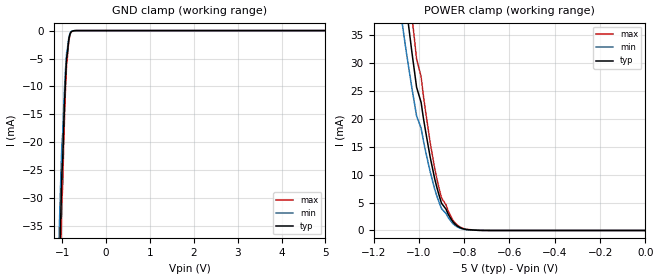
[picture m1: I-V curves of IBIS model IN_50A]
| TEXAS INSTRUMENTS INCORPORATED
| Standard Linear and Logic Group / High Volume Linear
| IBIS Model of TPD6E05U06
| Six Channel ESD Protection Device
| This file contains package information for the following:
|  UQFN 14-pin  package as [Component] TPD6E05U06RVZR
| This device can be powered at the following Vccs:
|  5 volt Vcc
[IBIS Ver]   3.2
[Comment char]  |_char
[File Name]   tpd6e05u06.ibs
[File Rev]   1.1
[Date]   12/10/2015
[Source]   Data created from TI-SPICE simulations at TI-SLL/HVL.
   The following is an IBIS list for the TPD4E05U06.
   Please contact sllibis@ti.com with questions and
   comments concerning SLL IBIS models.
[Notes]   Revision_History:
|  Rev 1.1   12/10/2015
|  - c comp values revised per PL's request
|  Rev 1.0 05/02/2013
[Disclaimer]
| This model is designed as an aid for customers of Texas Instruments.
| TI and its licensors and suppliers make no warranties, either expressed
| or implied, with respect to this  model, including the warranties of
| merchantability or fitness for a particular purpose. The model is
| provided solely on an "as is" basis. The entire risk as to its quality
| and performance is with the customer.
[Copyright]
| (C) Copyright 2013 Texas Instruments Incorporated. All rights reserved.
| Component TPD6E05U06RVZR
[Component]   TPD6E05U06RVZR
[Manufacturer]   Texas Instruments, Inc.
[Package]
|   typ   min   max
R_pkg   0.02313   0.00041   0.06326
L_pkg   0.30296nH   0.01585nH   1.03943nH
C_pkg   0.16466pF   0.07425pF   0.45674pF
[Pin]   signal_name   model_name   R_pin   L_pin   C_pin
1   NC   NC   0.00041   0.01757nH   0.07425pF
2   NC   NC   0.00041   0.01662nH   0.09156pF
3   NC   NC   0.00041   0.01593nH   0.1079pF
4   NC   NC   0.00041   0.01585nH   0.10796pF
5   GND   GND   0.00041   0.01593nH   0.45674pF
6   NC   NC   0.00041   0.01662nH   0.09156pF
7   NC   NC   0.00041   0.01755nH   0.07457pF
8   D3-   IN_50A   0.04552   1.03943nH   0.11983pF
9   D3+   IN_50A   0.06326   0.78248nH   0.16047pF
10   GND   GND   0.00041   0.01593nH   0.45674pF
11   D2-   IN_50A   0.04317   0.49796nH   0.1521pF
12   D2+   IN_50A   0.04311   0.49721nH   0.15259pF
13   D1-   IN_50A   0.04898   0.58006nH   0.14353pF
14   D1+   IN_50A   0.04173   0.71227nH   0.11545pF
| Models and submodels in the file (1): IN_50A (Input)
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[Model]   IN_50A
Model_type  Input
Vinl=0
Vinh=5
| variable   typ   min   max
C_comp   0.31pF   0.21pF   0.61pF
[Temperature Range]   40   100   -40
| Ambient temperature   25   85   -40
[Voltage range]   5   5   5
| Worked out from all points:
|   GND clamp passes 1 mA (typ) near -0.84 V on its own axis
|   POWER clamp passes 1 mA (typ) near -0.84 V on its own axis
[GND Clamp]
| IN_50A
| Voltage   I(typ)   I(min)   I(max)
-5V       -1.23A     -985mA     -1.48A
-1.07V    -45.16mA   -36.1mA    -54.2mA
-1.05V    -38.18mA   -30.5mA    -45.8mA
-1.03V    -31.67mA   -25.3mA    -38mA
-1.02V    -28.68mA   -22.9mA    -34.4mA
-1.01V    -25.62mA   -20.5mA    -30.7mA
-990mV    -22.9mA    -18.3mA    -27.5mA
-950mV    -13.12mA   -10.5mA    -15.7mA
-900mV    -4.871mA   -3.9mA     -5.84mA
-850mV    -1.552mA   -1.24mA    -1.86mA
-790mV    -170.1uA   -136uA     -204uA
5V        247pA      198pA      296pA
[POWER Clamp]
| IN_50A
|Voltage   I(typ)   I(min)   I(max)
-5V       1.23A      985mA      1.48A
-1.07V    45.16mA    36.1mA     54.2mA
-1.05V    38.18mA    30.5mA     45.8mA
-1.03V    31.67mA    25.3mA     38mA
-1.02V    28.68mA    22.9mA     34.4mA
-1.01V    25.62mA    20.5mA     30.7mA
-990mV    22.9mA     18.3mA     27.5mA
-950mV    13.12mA    10.5mA     15.7mA
-920mV    7.63mA     6.1mA      9.16mA
-900mV    4.871mA    3.9mA      5.84mA
-830mV    797.3uA    638uA      957uA
0V        0A         0A         0A
